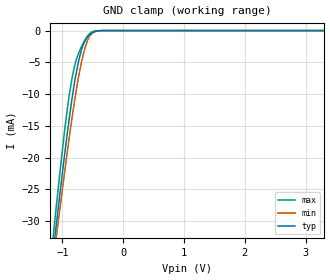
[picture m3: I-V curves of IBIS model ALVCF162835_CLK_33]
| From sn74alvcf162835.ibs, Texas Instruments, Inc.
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[Model]   ALVCF162835_CLK_33
Model_type  Input
Vinl=0.8
Vinh=2.0
| variable   typ   min   max
C_comp   2.41pF   1.96pF   3.01pF
[Temperature Range]   40   100   -40
| Ambient temperature   25   85   -40
[Voltage range]   3.3   3   3.6
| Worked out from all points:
|   GND clamp passes 1 mA (typ) near -0.58 V on its own axis
[GND Clamp]
| ALVCF162835_CLK_33
|   Voltage   I(typ)   I(min)   I(max)
-3.3V     -233.4mA   -219.5mA   -250mA
-1.165V   -35.98mA   -37.59mA   -33.63mA
-1.14V    -33.87mA   -35.64mA   -31.31mA
-1.115V   -31.78mA   -33.7mA    -29.01mA
-1.09V    -29.7mA    -31.78mA   -26.72mA
-935mV    -17.33mA   -20.21mA   -13.52mA
-815mV    -9.03mA    -12mA      -6.225mA
-750mV    -5.573mA   -8.121mA   -3.977mA
-675mV    -2.707mA   -4.493mA   -2.304mA
-590mV    -1.074mA   -1.656mA   -901.9uA
-515mV    -393.6uA   -466.9uA   -227.6uA
3.3V      193.8pA    964.4pA    46.32pA
